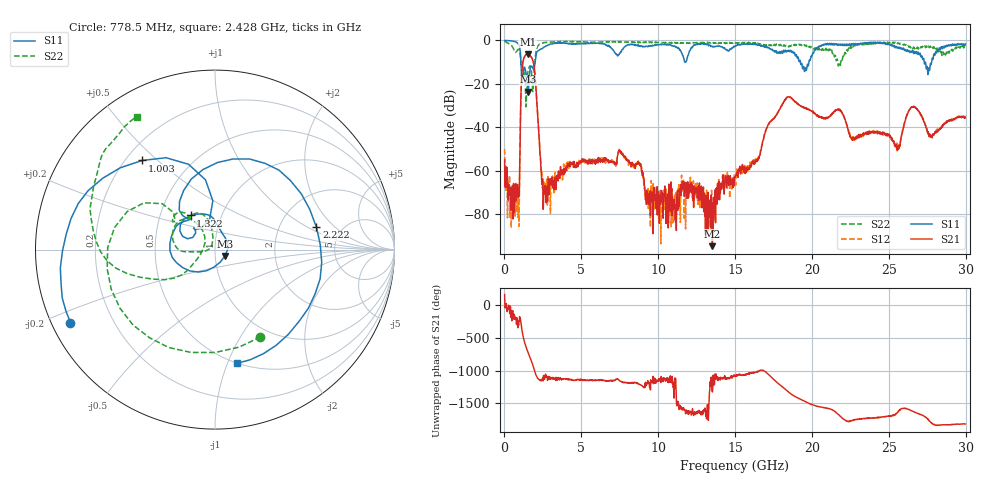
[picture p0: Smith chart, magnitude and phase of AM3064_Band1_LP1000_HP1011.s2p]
# Hz S DB R 50.0
!freq dBS11 angS11 dBS21 angS21 dBS12 angS12 dBS22 angS22
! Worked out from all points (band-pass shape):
!   1600 points, 10 MHz to 29.98 GHz, reference 50 ohm
!   highest |S21| = -6.29 dB at 1.51 GHz (marker M1); lowest = -94.9 dB at 13.52 GHz (marker M2)
!   |S21| within 3 dB of the highest: 1.219 GHz to 1.846 GHz (626.5 MHz wide, 40.9 % of centre)
!   lowest |S11| = -23.7 dB at 1.547 GHz (marker M3), VSWR 1.14, Z = 55.7 - j4 ohm
!   |S11| at or under -10 dB: 1.071 GHz to 1.988 GHz (917.6 MHz wide, 60 % of centre); 19.24 GHz to 19.81 GHz (564 MHz wide, 2.89 % of centre); 27.38 GHz to 27.78 GHz (404.9 MHz wide, 1.47 % of centre)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
!   |S22| runs from -30.6 to -0.4 dB; largest |S21 - S12| = 0.007
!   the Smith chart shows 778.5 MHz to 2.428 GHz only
!   S11 on the Smith chart (normalised r, x): 778.5 MHz: 0.05, -0.24; 1.003 GHz: 0.26, +0.45; 1.322 GHz: 0.71, +0.29; 2.222 GHz: 3.25, +1.22; 2.428 GHz: 0.50, -1.08
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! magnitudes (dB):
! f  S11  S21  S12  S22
! 10 MHz  -0.1  -54.9  -50.1  -0.4
! 778.5 MHz  -0.9  -69.3  -71.7  -5.2
! 1.003 GHz  -3.9  -51.9  -51.3  -5.5
! 1.172 GHz  -15.9  -11.3  -11.2  -11.6
! 1.322 GHz  -12.6  -7.4  -7.3  -14.9
! 1.51 GHz  -22.1  -6.3  -6.3  -15.3
! 1.547 GHz  -23.7  -6.5  -6.3  -13.8
! 1.903 GHz  -13.3  -10.9  -10.9  -16.0
! 2.222 GHz  -4.7  -41.5  -41.2  -2.2
! 2.428 GHz  -3.8  -65.3  -60.5  -1.3
! 5.015 GHz  -1.5  -55.6  -55.9  -0.6
! 7.564 GHz  -5.3  -52.2  -51.3  -0.6
! 10 GHz  -2.0  -72.0  -73.3  -0.9
! 13.52 GHz  -3.0  -94.9  -81.6  -1.3
! 15 GHz  -2.8  -63.0  -63.6  -1.4
! 18.36 GHz  -5.3  -26.4  -26.5  -2.8
! 19.99 GHz  -7.4  -32.7  -32.6  -3.1
! 25 GHz  -1.5  -43.9  -43.7  -1.1
! 25.63 GHz  -3.5  -50.1  -48.1  -1.2
! 26.59 GHz  -5.4  -30.7  -30.6  -3.3
! 27.56 GHz  -15.2  -42.2  -42.8  -2.7
! 29.98 GHz  -1.7  -35.7  -35.2  -3.2
